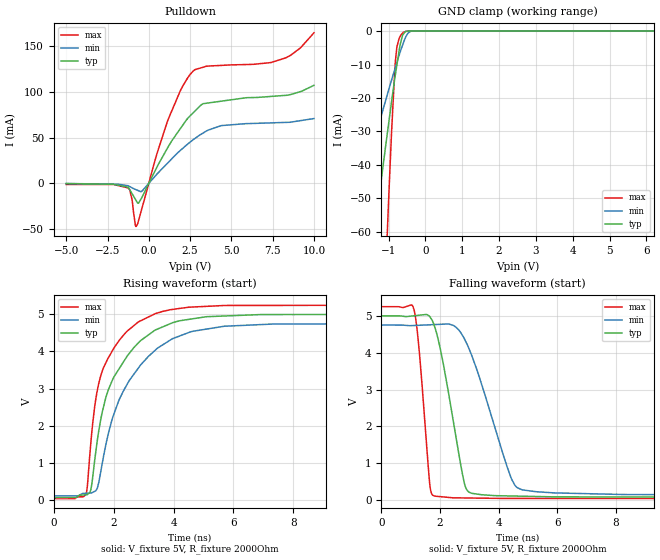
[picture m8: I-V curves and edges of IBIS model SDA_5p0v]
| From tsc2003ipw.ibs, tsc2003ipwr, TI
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|   SDA_5p0v
[Model]   SDA_5p0v
Model_type   I/O_open_drain
Polarity   Non-Inverting
Enable   Active-High
Vinl = 1.5
Vinh = 3.5
Vmeas = 2.5
Vref = 2.5
Cref = 1pF
Rref = 50
|   typ   min   max
C_comp   0.463pF   0.359pF   0.528pF
[Voltage Range]   5   4.75   5.25
[Temperature Range]   27   85   -40
[Pullup Reference]   5   4.75   5.25
[Pulldown Reference]   0   0   0
[Power Clamp Reference]   5   4.75   5.25
[GND Clamp Reference]   0   0   0
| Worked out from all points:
|   slope of the pulldown table from 0 to 0.75 V, typ, clamps not added: 28.6 ohm
|   GND clamp passes 1 mA (typ) near -0.60 V on its own axis
|   falling waveform, V_fixture 5V, R_fixture 2000Ohm: 20-80 % time 651ps typ, 1.1ns min, 310ps max; typ from 5 V to 0.065 V
|   rising waveform, V_fixture 5V, R_fixture 2000Ohm: 20-80 % time 1.22ns typ, 1.48ns min, 919ps max; typ from 0.064 V to 5 V
[Pulldown]
|   Voltage   I(typ)   I(min)   I(max)
-5V       -311.5uA   -230.6uA   -1.245mA
-1.235V   -4.513mA   -2.707mA   -5.138mA
-1.01V    -11.38mA   -4.986mA   -18.17mA
-774.9mV  -18.54mA   -6.94mA    -47.3mA
-620.1mV  -21.7mA    -8.138mA   -40.75mA
1.142V    38.84mA    22.14mA    68.42mA
1.916V    59.93mA    35.98mA    101.4mA
2.681V    77mA       47.56mA    122.6mA
3.284V    87.02mA    54.91mA    126.9mA
4.371V    89.72mA    62.97mA    128.8mA
8.288V    96.12mA    66.57mA    137mA
10V       107.1mA    70.76mA    164.5mA
[GND Clamp]
|   Voltage   I(typ)   I(min)   I(max)
-5V       -381.2mA   -176.9mA   -1.217A
-2.135V   -126.2mA   -62.07mA   -376.8mA
-1.535V   -73.46mA   -38.35mA   -201.6mA
-1.246V   -48.45mA   -27.07mA   -118.7mA
-1.076V   -33.98mA   -20.57mA   -71.36mA
-1.01V    -28.54mA   -18.04mA   -53.26mA
-919.2mV  -21.08mA   -14.65mA   -30.16mA
-813.4mV  -12.87mA   -10.79mA   -8.771mA
-714.2mV  -5.83mA    -7.219mA   -2.204mA
-543.3mV  -134.4uA   -1.984mA   -181.5uA
-331.9mV  -2.434uA   -9.442uA   -2.756uA
10V       0A         0A         0A
[POWER Clamp]
|   Voltage   I(typ)   I(min)   I(max)
-5V       0A         0A         0A
0V        0A         0A         0A
10V       0A         0A         0A
[Ramp]
R_load = 2000
|   typ   min   max
dV/dt_r   2.96158/1.21767e-009   2.78437/1.48073e-009   3.12914/9.14978e-010
dV/dt_f   2.96102/6.50489e-010   2.78125/1.10061e-009   3.12913/3.09392e-010
[Falling Waveform]
V_fixture = 5V
V_fixture_min = 4.75V
V_fixture_max = 5.25V
R_fixture = 2000Ohm
C_fixture = 0F
|   Time   V(typ)   V(min)   V(max)
0s        5V         4.75V      5.25V
1.116ns   5.002V     4.738V     5.175V
1.3ns     5.018V     4.744V     4.005V
1.654ns   4.98V      4.757V     432.8mV
1.804ns   4.746V     4.763V     108.2mV
2.827ns   479.6mV    4.389V     55.15mV
3.074ns   184.5mV    3.949V     52.71mV
4.408ns   108.8mV    640.3mV    41.59mV
4.794ns   102.6mV    278mV      41.43mV
20.78ns   64.97mV    114.6mV    34.79mV
[Rising Waveform]
V_fixture = 5V
V_fixture_min = 4.75V
V_fixture_max = 5.25V
R_fixture = 2000Ohm
C_fixture = 0F
|   Time   V(typ)   V(min)   V(max)
0s        64.02mV    109.4mV    34.76mV
1.078ns   138.7mV    181.4mV    168.3mV
1.241ns   289.6mV    188.4mV    1.58V
1.429ns   1.464V     280.7mV    2.848V
1.736ns   2.754V     1.48V      3.689V
2.16ns    3.506V     2.656V     4.268V
3.393ns   4.577V     4.037V     5.017V
4.551ns   4.866V     4.521V     5.19V
5.687ns   4.952V     4.676V     5.235V
20.78ns   5V         4.75V      5.25V
